//{{V2}}
FUNCTION FC15
TITLE=Write UInt16 SDO
//*****************************************************************************
//* maxon motor ag
//* R&D
//* all rights reserved
//*****************************************************************************
//* Summary:  Write an UInt16 object via SDO
//*
//* Remarks:
//*
//* Created under: STEP7 REV5.2+SP1
//*****************************************************************************
//* History:
//* 18.05.2004 | INA   first release
//*
//*
//*****************************************************************************


AUTHOR:INA
FAMILY:SDO
NAME:WrUInt16
VERSION:00.01


VAR_INPUT
       NodeID:BYTE
       Index:DWORD
       SubIndex:DWORD
       ValueIn:WORD
END_VAR

VAR_OUTPUT
       RET_VAL:BOOL //Done
       Err:BOOL //True = Error detected
       ErrNo:DINT //Error number (CAN or/and VIPA!)
END_VAR

VAR_IN_OUT
END_VAR

VAR_TEMP
       xBusy:BOOL //The write job is not yet completed
       xCanOpenError:DWORD //Return value from SDO transfer
       xRetValue:WORD //VIPA Error
       xValueIn:WORD
END_VAR
BEGIN

NETWORK
TITLE=
//{{a}}

// SDO Write UInt16

       R    #RET_VAL                     // Done
       R    #Err
       L    0
       T    #ErrNo

       L    #ValueIn
       T    #xValueIn

sfc   :NOP  0

       CALL SFC219
         Request:=TRUE
         Slot_Master:=B#16#00
         NodeID:=#NodeID
         Transfertyp:=B#16#2B            // Write
         Index:=#Index
         Subindex:=#SubIndex
         CanOpenError:=#xCanOpenError
         RetVal:=#xRetValue
         Busy:=#xBusy
         DataBuffer:=P#L 8.0 WORD 1

       L    1
       U    #xBusy
       SPB  sfc

       S    #RET_VAL

       L    W#16#F021
       L    #xRetValue
       <I
       SPBN ok                           // jump if RetValue lower than 0xF021
       L    W#16#F028
       L    #xRetValue
       >I
       SPB  errV                         // jump if xRetValue between 0xF021 and 0xF028

       L    0
       L    #xCanOpenError
       <>D
       SPB  errC                         // jump if CAN error

ok    :NOP  0
       R    #Err
       SPA  end

errC  :NOP  0                            // CANopen error
       S    #Err
       L    #xCanOpenError
       TAD
       T    #ErrNo
       SPA  end

errV  :NOP  0                            // VIPA error
       S    #Err
       L    0
       T    #ErrNo
       L    #xRetValue                   // RetVal
       T    #ErrNo

end   :NOP  0
END_FUNCTION
